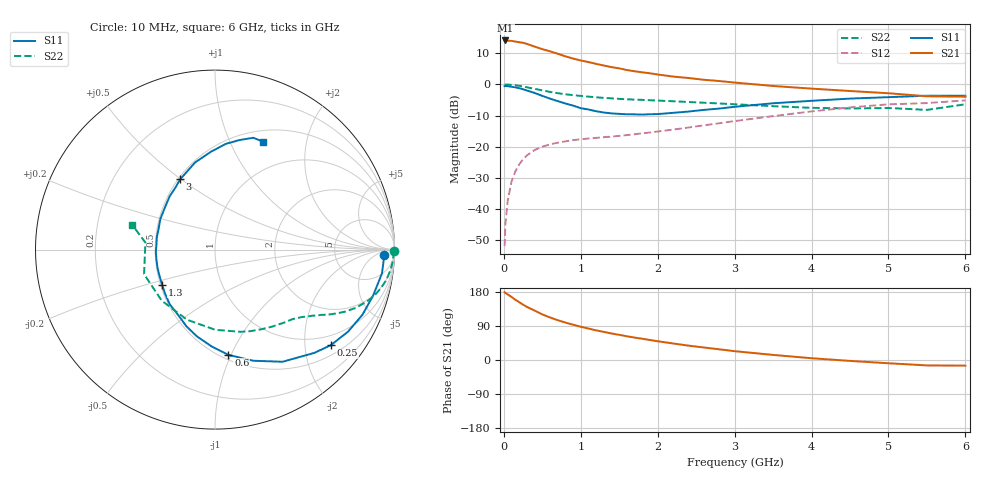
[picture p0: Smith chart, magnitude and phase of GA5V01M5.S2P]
! Infineon Technologies  Discrete & RF Semiconductors
! BF775
! Si NPN RF Bipolar Junction Transistor in SOT23
! VCE = 5 V  IC = 1.5 mA
! Common Emitter S-Parameters:  May  1996
# GHz  S  MA  R  50
!  f  S11  S21  S12  S22
! GHz  MAG  ANG  MAG  ANG  MAG  ANG  MAG  ANG
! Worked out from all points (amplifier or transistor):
!   36 points, 10 MHz to 6 GHz, reference 50 ohm
!   highest |S21| = 14.2 dB at 20 MHz (marker M1)
!   |S21| within 3 dB of that: start of sweep to 529.1 MHz
!   unconditionally stable (mu >= 1): 1.301 GHz to 3.638 GHz; 5.376 GHz to 5.731 GHz
!   at 250 MHz: K = 0.24, MSG = 18.7 dB, |S12| = -24.1 dB
!   at 1.4 GHz: K = 1.05, MAG = 9.8 dB, |S12| = -16.8 dB
!   at 6 GHz: K = 0.98, MSG = 0.6 dB, |S12| = -5.1 dB
!   S11 on the Smith chart (normalised r, x): 10 MHz: 26, -13; 250 MHz: 0.73, -2.60; 600 MHz: 0.54, -0.98; 1.3 GHz: 0.51, -0.23; 3 GHz: 0.51, +0.50; 6 GHz: 0.63, +1.34
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0.01  0.9402 -1.7  5.084 178.8  0.0025 92.8  0.9999 -0.6
0.02  0.9421 -3.3  5.103 177.0  0.0056 88.4  0.9944 -1.4
0.05  0.9397 -8.1  5.04 173.1  0.0134 84.9  0.994 -3.4
0.1  0.917 -16.4  5.028 166.4  0.0274 80.1  0.9836 -6.8
0.15  0.8979 -23.9  4.895 158.9  0.0399 75.0  0.9686 -10.2
0.25  0.8368 -39.5  4.684 146.0  0.0626 67.2  0.9261 -15.9
0.3  0.7985 -46.1  4.491 140.1  0.0722 63.7  0.8994 -18.4
0.4  0.7297 -58.9  4.066 130.4  0.088 57.7  0.8501 -22.4
0.5  0.655 -71.0  3.697 120.3  0.0998 52.5  0.803 -25.5
0.6  0.5915 -82.7  3.415 112.3  0.1087 48.8  0.7596 -28.0
0.8  0.4941 -101.7  2.835 98.8  0.1215 44.0  0.6946 -31.6
0.9  0.4567 -110.3  2.608 93.1  0.1273 42.7  0.6735 -33.0
1.1  0.3953 -129.7  2.29 82.9  0.135 41.2  0.6368 -35.8
1.3  0.3536 -146.6  2.016 74.1  0.1417 41.4  0.608 -38.3
1.7  0.3301 -177.8  1.63 59.2  0.1579 43.4  0.5702 -44.0
2.2  0.3493 150.6  1.339 43.6  0.1877 46.3  0.5369 -52.7
3  0.4369 116.4  1.073 23.3  0.2572 46.7  0.48 -72.6
3.5  0.4979 102.9  0.945 13.4  0.3096 43.6  0.447 -89.8
4.5  0.5921 84.2  0.784 -2.4  0.4275 32.1  0.4112 -136.2
5  0.6244 77.6  0.722 -8.6  0.4785 24.3  0.4182 -160.9
5.5  0.6586 71.1  0.645 -14.3  0.5015 15.3  0.3897 174.2
6  0.658 65.8  0.635 -14.9  0.5539 10.6  0.4796 163.5
